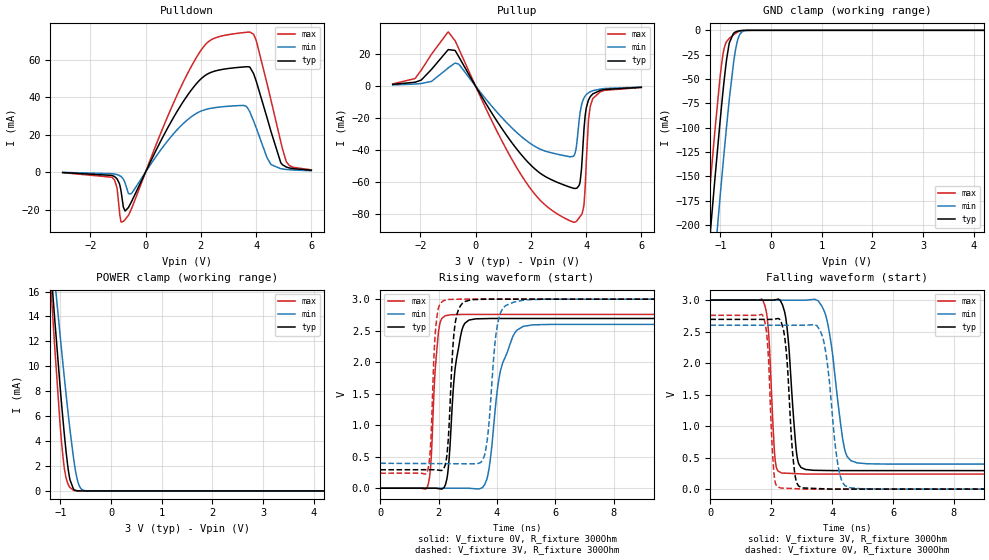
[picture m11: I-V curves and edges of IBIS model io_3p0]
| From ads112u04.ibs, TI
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|   io_3p0 Model
[Model]   io_3p0
Model_type   I/O
Polarity   Non-Inverting
Enable   Active-Low
Vinl = 0.9
Vinh = 2.1
Vmeas = 1.5
Vref = 0
Cref = 2pF
Rref = 100000
|   typ   min   max
C_comp   1.45093E-12   1.45086E-12   1.4642E-12
|C_comp_pullup   1.23493E-12   1.23488E-12   1.24627E-12
|C_comp_pulldown   1.15247E-12   1.14193E-12   1.21789E-12
[Model spec]
|subparameter
Vinl   0.9   0.8997   0.9003
Vinh   2.1   2.0993   2.1007
| Where Nom  PVT is Nominal Process, 3.0V, 27C
|   Fast PVT is Strong Process,  3.001V, -40C
|   Slow PVT is Weak Process,   2.999, 125C
[Voltage Range]   3   2.999   3.001
[Temperature Range]   27   125   -40
[Pullup Reference]   3   2.999   3.001
[Pulldown Reference]   0   -0   -0
[Power Clamp Reference]   3   2.999   3.001
[GND Clamp Reference]   0   0   0
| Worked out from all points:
|   slope of the pulldown table from 0 to 0.45 V, typ, clamps not added: 32.9 ohm
|   slope of the pullup table from 0 to 0.45 V, typ, clamps not added: 34.5 ohm
|   GND clamp passes 1 mA (typ) near -0.67 V on its own axis
|   POWER clamp passes 1 mA (typ) near -0.82 V on its own axis
|   falling waveform, V_fixture 3V, R_fixture 300Ohm: 20-80 % time 240ps typ, 401ps min, 165ps max; typ from 3 V to 0.293 V
|   rising waveform, V_fixture 0V, R_fixture 300Ohm: 20-80 % time 283ps typ, 495ps min, 188ps max; typ from 0 V to 2.69 V
|   rising waveform, V_fixture 3V, R_fixture 300Ohm: 20-80 % time 189ps typ, 275ps min, 147ps max; typ from 0.293 V to 3 V
|   falling waveform, V_fixture 0V, R_fixture 300Ohm: 20-80 % time 210ps typ, 330ps min, 153ps max; typ from 2.69 V to 0 V
[Pulldown]
|   Voltage   I(typ)   I(min)   I(max)
-3V       -273.9uA   -170.1uA   -318.1uA
-1.209V   -1.837mA   -882.5uA   -2.873mA
-1.038V   -3.532mA   -1.358mA   -8.235mA
-948mV    -6.156mA   -1.851mA   -20.53mA
-804mV    -18.75mA   -3.789mA   -26.31mA
-525mV    -16.24mA   -11.64mA   -20.1mA
1.977V    49.29mA    32.32mA    64.32mA
3.75V     56.09mA    32.76mA    74.65mA
3.993V    48.97mA    24.06mA    70.62mA
4.542V    21.51mA    3.966mA    38.21mA
5.091V    2.699mA    1.387mA    5.655mA
6V        980.2uA    687.2uA    1.154mA
[GND Clamp]
|   Voltage   I(typ)   I(min)   I(max)
-3V       -1.375A    -1.451A    -1.328A
-1.317V   -280.6mA   -360.8mA   -230.1mA
-1.164V   -185.9mA   -265.9mA   -135.8mA
-1.11V    -153.4mA   -233mA     -103.9mA
-1.011V   -96.03mA   -173.8mA   -50.2mA
-930mV    -53.24mA   -127.2mA   -19.27mA
-876mV    -29.29mA   -97.54mA   -11.4mA
-822mV    -12.54mA   -69.63mA   -8.135mA
-696mV    -1.531mA   -18.49mA   -2.905mA
-615mV    -375.9uA   -4.123mA   -864uA
-480mV    -15.03uA   -143.5uA   -25.62uA
6V        0A         0A         0A
[Pullup]
|   Voltage   I(typ)   I(min)   I(max)
-3V       1.091mA    745.1uA    1.366mA
-2.19V    2.436mA    1.303mA    4.757mA
-984mV    22.89mA    11.5mA     33.86mA
-615mV    18.63mA    13.82mA    23.65mA
1.779V    -45.45mA   -33.32mA   -59.05mA
3.561V    -64.06mA   -43.66mA   -85.26mA
3.642V    -64.04mA   -38.75mA   -84.77mA
3.786V    -59.67mA   -16.42mA   -81.65mA
3.921V    -27.83mA   -7.527mA   -74.85mA
4.092V    -8.532mA   -4.111mA   -20.65mA
4.245V    -4.856mA   -2.861mA   -7.757mA
6V        -745.8uA   -590.3uA   -837.5uA
[POWER Clamp]
|   Voltage   I(typ)   I(min)   I(max)
-3V       122.6mA    105.5mA    143.3mA
-1.182V   17.52mA    19.99mA    16.04mA
-1.164V   16.55mA    19.21mA    14.87mA
-1.128V   14.62mA    17.65mA    12.57mA
-1.11V    13.67mA    16.87mA    11.43mA
-1.002V   8.185mA    12.32mA    5.129mA
-930mV    4.865mA    9.401mA    2.037mA
-840mV    1.557mA    5.946mA    466.4uA
-741mV    140.7uA    2.651mA    45.51uA
-633mV    6.443uA    467.2uA    1.704uA
-498mV    123.3nA    13.64uA    2.411nA
6V        0A         0A         0A
[Ramp]
R_load = 300
|   typ   min   max
dV/dt_r   1.6162/2.82986e-10   1.56008/4.92338e-10   1.65491/1.87801e-10
dV/dt_f   1.62405/2.39337e-10   1.56183/3.99698e-10   1.65761/1.64248e-10
[Falling Waveform]
V_fixture = 3V
V_fixture_min = 2.999V
V_fixture_max = 3.001V
R_fixture = 300Ohm
C_fixture = 0F
|   Time   V(typ)   V(min)   V(max)
0s        3V         2.999V     3.001V
1.73ns    2.999V     2.998V     2.995V
2.132ns   3.005V     2.998V     460.9mV
2.346ns   2.947V     2.998V     256.6mV
2.842ns   543.5mV    2.998V     245.6mV
3.126ns   312.4mV    2.998V     239.3mV
3.768ns   296.5mV    2.791V     239.1mV
4.408ns   294.3mV    641.4mV    239.1mV
4.82ns    294.3mV    417.3mV    239.1mV
50ns      293.2mV    396mV      238.3mV
[Rising Waveform]
V_fixture = 0V
V_fixture_min = 0V
V_fixture_max = 0V
R_fixture = 300Ohm
C_fixture = 0F
|   Time   V(typ)   V(min)   V(max)
0s        -294.4nV   -687.1nV   -468.3nV
1.605ns   731.4uV    420.1uV    7.68mV
2.003ns   -6.626mV   524.6uV    2.502V
2.414ns   862.7mV    632.2uV    2.752V
2.572ns   1.924V     673.9uV    2.754V
2.899ns   2.617V     759.4uV    2.758V
3.644ns   2.691V     129.7mV    2.758V
4.181ns   2.693V     1.966V     2.758V
5.216ns   2.693V     2.592V     2.758V
50ns      2.694V     2.6V       2.758V
[Rising Waveform]
V_fixture = 3V
V_fixture_min = 2.999V
V_fixture_max = 3.001V
R_fixture = 300Ohm
C_fixture = 0F
|   Time   V(typ)   V(min)   V(max)
0s        293.2mV    396mV      238.3mV
1.596ns   293.8mV    391.5mV    242.8mV
1.946ns   289.8mV    390.5mV    2.735V
2.346ns   893.6mV    389.3mV    2.995V
2.52ns    2.425V     388.9mV    2.997V
2.745ns   2.893V     388.2mV    3V
3.523ns   2.997V     461.1mV    3V
4.065ns   2.999V     2.695V     3V
4.97ns    2.999V     2.989V     3V
50ns      3V         2.999V     3.001V
[Falling Waveform]
|Gnd
V_fixture = 0V
V_fixture_min = 0V
V_fixture_max = 0V
R_fixture = 300Ohm
C_fixture = 0F
|   Time   V(typ)   V(min)   V(max)
0s        2.694V     2.6V       2.758V
1.719ns   2.693V     2.6V       2.759V
2.091ns   2.696V     2.6V       253.3mV
2.305ns   2.671V     2.6V       18.49mV
2.769ns   268.3mV    2.6V       8.163mV
3.029ns   19.84mV    2.6V       2.384mV
3.692ns   6.506mV    2.408V     809.5uV
4.218ns   1.064mV    317.7mV    809.1uV
4.601ns   1.064mV    21.43mV    808.8uV
50ns      -302.3nV   -7.409nV   -234.3nV
